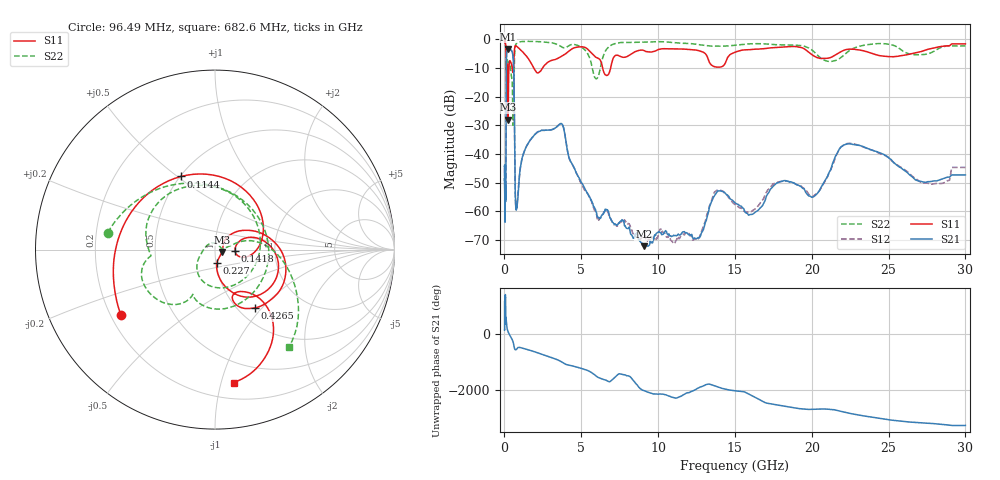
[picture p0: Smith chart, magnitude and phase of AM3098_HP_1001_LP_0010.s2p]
! Date/Time: Thu, Feb 28, 2019 8:40 AM
! Network Analyzer: Agilent Technologies E8364B Rev: A.07.50.67
! Sweep from 0.010 to 30.000 GHz, 1601 Points, Sweep Type: LOG
! Power Supply: 5.023 V, 0.002 A
# Hz S DB R 50
!freq MagS11 AngS11 MagS21 AngS21 MagS12 AngS12 MagS22 AngS22
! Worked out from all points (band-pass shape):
!   1601 points, 10 MHz to 30 GHz, reference 50 ohm
!   highest |S21| = -3.33 dB at 239.9 MHz (marker M1); lowest = -72.2 dB at 9.072 GHz (marker M2)
!   |S21| within 3 dB of the highest: 129.4 MHz to 566.5 MHz (437.1 MHz wide, 126 % of centre)
!   lowest |S11| = -28.0 dB at 237.5 MHz (marker M3), VSWR 1.08, Z = 53.9 - j1.37 ohm
!   |S11| at or under -10 dB: 198.7 MHz to 290.3 MHz (91.62 MHz wide, 37.5 % of centre); 1.909 GHz to 2.476 GHz (567.4 MHz wide, 25.9 % of centre); 6.39 GHz to 6.912 GHz (521.5 MHz wide, 7.84 % of centre)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
!   |S22| runs from -30.0 to -0.6 dB; largest |S21 - S12| = 0.011
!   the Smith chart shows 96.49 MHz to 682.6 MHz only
!   S11 on the Smith chart (normalised r, x): 96.49 MHz: 0.24, -0.30; 114.4 MHz: 0.50, +0.51; 141.8 MHz: 1.25, -0.02; 227 MHz: 1.01, -0.15; 426.5 MHz: 1.19, -0.91; 682.6 MHz: 0.32, -1.10
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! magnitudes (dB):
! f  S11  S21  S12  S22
! 10 MHz  -0.3  -44.5  -46.7  -0.6
! 38.04 MHz  -0.5  -59.6  -58.6  -0.8
! 96.49 MHz  -3.9  -45.3  -44.2  -4.4
! 114.4 MHz  -6.9  -16.6  -16.6  -10.5
! 141.8 MHz  -19.0  -4.6  -4.6  -11.0
! 144.7 MHz  -18.9  -4.5  -4.4  -10.6
! 185.8 MHz  -8.6  -3.9  -3.9  -7.1
! 227 MHz  -22.4  -3.4  -3.3  -8.8
! 237.5 MHz  -28.0  -3.3  -3.3  -8.9
! 239.9 MHz  -27.7  -3.3  -3.3  -8.9
! 426.5 MHz  -8.1  -3.7  -3.7  -11.8
! 550.5 MHz  -11.5  -5.6  -5.5  -28.4
! 617.6 MHz  -6.2  -13.5  -13.4  -13.7
! 682.6 MHz  -2.5  -45.9  -46.4  -3.3
! 785.3 MHz  -2.4  -59.3  -58.3  -1.4
! 2.084 GHz  -11.5  -32.7  -32.6  -0.7
! 3.723 GHz  -5.8  -29.4  -29.4  -2.6
! 7.926 GHz  -6.1  -65.8  -63.6  -1.0
! 9.072 GHz  -3.8  -72.2  -68.3  -0.9
! 20.1 GHz  -5.6  -55.0  -54.8  -4.1
! 22.56 GHz  -3.4  -36.5  -36.3  -3.5
! 30 GHz  -1.5  -47.3  -44.7  -2.3
